FUNCTION FC 20 : VOID
TITLE =CICLO AUTOMATICO
VERSION : 0.1

BEGIN
NETWORK
TITLE =START CICLO AUTOMATICO ASPO
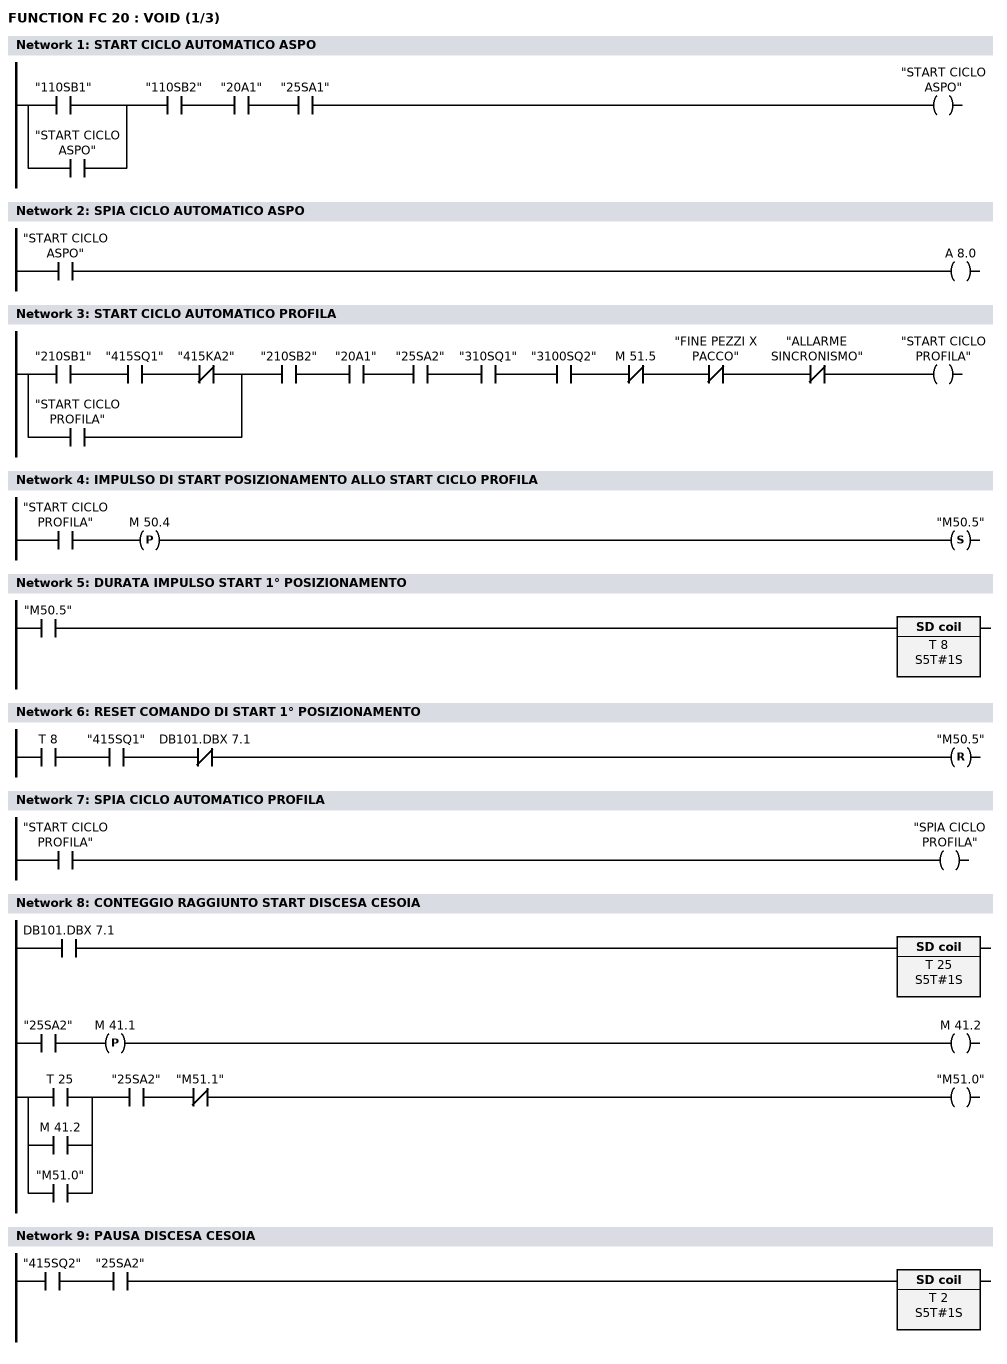
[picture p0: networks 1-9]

      U(    ;
      O     "110SB1";
      O     "START CICLO ASPO";
      )     ;
      U     "110SB2";
      U     "20A1";
      U     "25SA1";
      =     "START CICLO ASPO";
NETWORK
TITLE =SPIA CICLO AUTOMATICO ASPO

      U     "START CICLO ASPO";
      =     A      8.0;
NETWORK
TITLE =START CICLO AUTOMATICO PROFILA

      U     "210SB1";
      U     "415SQ1";
      UN    "415KA2";
      O     "START CICLO PROFILA";
      U     "210SB2";
      U     "20A1";
      U     "25SA2";
      U     "310SQ1";
      U     "3100SQ2";
      UN    M     51.5;
      UN    "FINE PEZZI X PACCO";
      UN    "ALLARME SINCRONISMO";
      =     "START CICLO PROFILA";
NETWORK
TITLE =IMPULSO DI START POSIZIONAMENTO ALLO START CICLO PROFILA

      U     "START CICLO PROFILA";
      FP    M     50.4;
      S     "M50.5";
NETWORK
TITLE =DURATA IMPULSO START 1° POSIZIONAMENTO

      U     "M50.5";
      L     S5T#1S;
      SE    T      8;
NETWORK
TITLE =RESET COMANDO DI START 1° POSIZIONAMENTO

      U     T      8;
      U     "415SQ1";
      UN    DB101.DBX    7.1;
      R     "M50.5";
NETWORK
TITLE =SPIA CICLO AUTOMATICO PROFILA

      U     "START CICLO PROFILA";
      =     "SPIA CICLO PROFILA";
NETWORK
TITLE =CONTEGGIO RAGGIUNTO START DISCESA CESOIA

      U     DB101.DBX    7.1;
      L     S5T#1S;
      SE    T     25;

      U     "25SA2";
      FP    M     41.1;
      =     M     41.2;

      U     T     25;
      O     M     41.2;
      O     "M51.0";
      U     "25SA2";
      UN    "M51.1";
      =     "M51.0";
NETWORK
TITLE =PAUSA DISCESA CESOIA

      U     "415SQ2";
      U     "25SA2";
      L     S5T#1S;
      SE    T      2;
NETWORK
TITLE =CONTEGGIO N° PEZZI
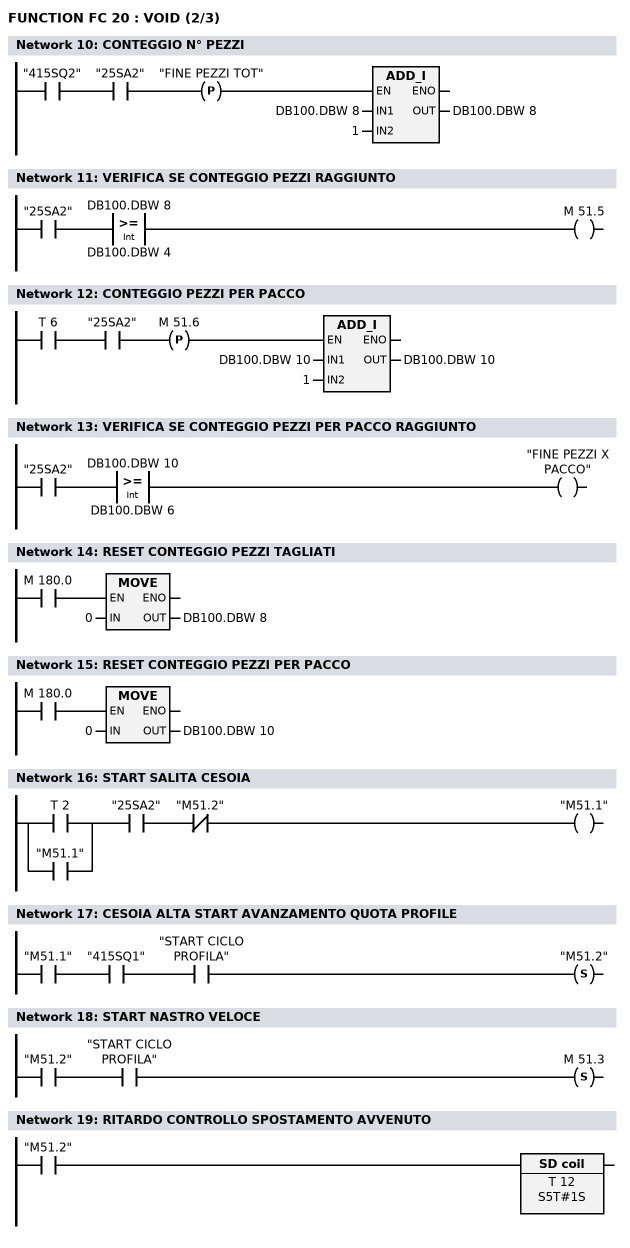
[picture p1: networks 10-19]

      U     "415SQ2";
      U     "25SA2";
      FP    "FINE PEZZI TOT";
      SPBNB _001;
      L     DB100.DBW    8;
      L     1;
      +I    ;
      T     DB100.DBW    8;
_001: NOP   0;
NETWORK
TITLE =VERIFICA SE CONTEGGIO PEZZI RAGGIUNTO

      U     "25SA2";
      U(    ;
      L     DB100.DBW    8;
      L     DB100.DBW    4;
      >=I   ;
      )     ;
      =     M     51.5;
NETWORK
TITLE =CONTEGGIO PEZZI PER PACCO

      U     T      6;
      U     "25SA2";
      FP    M     51.6;
      SPBNB _002;
      L     DB100.DBW   10;
      L     1;
      +I    ;
      T     DB100.DBW   10;
_002: NOP   0;
NETWORK
TITLE =VERIFICA SE CONTEGGIO PEZZI PER PACCO RAGGIUNTO
//
//
      U     "25SA2";
      U(    ;
      L     DB100.DBW   10;
      L     DB100.DBW    6;
      >=I   ;
      )     ;
      =     "FINE PEZZI X PACCO";
NETWORK
TITLE =RESET CONTEGGIO PEZZI TAGLIATI

      U     M    180.0;
      SPBNB _003;
      L     0;
      T     DB100.DBW    8;
_003: NOP   0;
NETWORK
TITLE =RESET CONTEGGIO PEZZI PER PACCO

      U     M    180.0;
      SPBNB _004;
      L     0;
      T     DB100.DBW   10;
_004: NOP   0;
NETWORK
TITLE =START SALITA CESOIA

      U(    ;
      O     T      2;
      O     "M51.1";
      )     ;
      U     "25SA2";
      UN    "M51.2";
      =     "M51.1";
NETWORK
TITLE =CESOIA ALTA START AVANZAMENTO QUOTA PROFILE

      U     "M51.1";
      U     "415SQ1";
      U     "START CICLO PROFILA";
      S     "M51.2";
NETWORK
TITLE =START NASTRO VELOCE

      U     "M51.2";
      U     "START CICLO PROFILA";
      S     M     51.3;
NETWORK
TITLE =RITARDO CONTROLLO SPOSTAMENTO AVVENUTO

      U     "M51.2";
      L     S5T#1S;
      SE    T     12;
NETWORK
TITLE =RESET START AVANZAMENTO A QUOTA
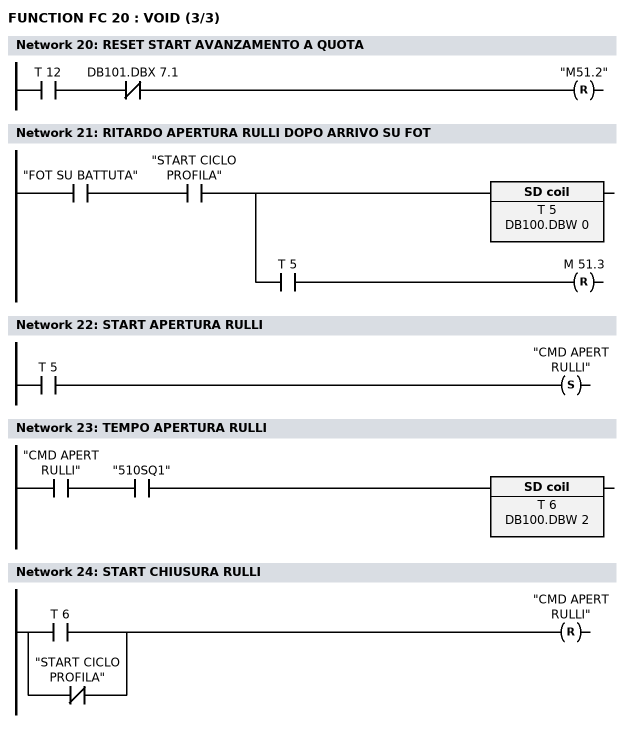
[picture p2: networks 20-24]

      U     T     12;
      UN    DB101.DBX    7.1;
      R     "M51.2";
NETWORK
TITLE =RITARDO APERTURA RULLI DOPO ARRIVO SU FOT

      U     "FOT SU BATTUTA";
      U     "START CICLO PROFILA";
      =     L      0.0;
      U     L      0.0;
      BLD   102;
      L     DB100.DBW    0;
      SE    T      5;
      U     L      0.0;
      U     T      5;
      R     M     51.3;
NETWORK
TITLE =START APERTURA RULLI

      U     T      5;
      S     "CMD APERT RULLI";
NETWORK
TITLE =TEMPO APERTURA RULLI

      U     "CMD APERT RULLI";
      U     "510SQ1";
      L     DB100.DBW    2;
      SE    T      6;
NETWORK
TITLE =START CHIUSURA RULLI

      O     T      6;
      ON    "START CICLO PROFILA";
      R     "CMD APERT RULLI";
END_FUNCTION

